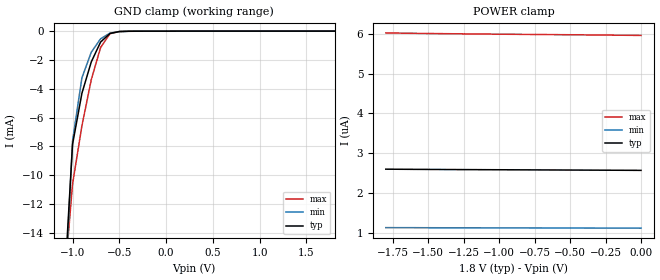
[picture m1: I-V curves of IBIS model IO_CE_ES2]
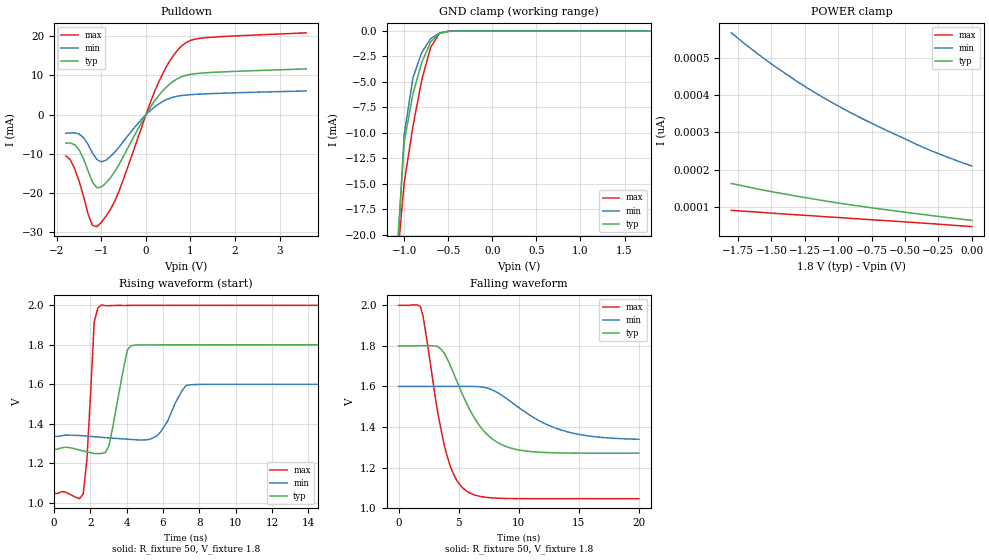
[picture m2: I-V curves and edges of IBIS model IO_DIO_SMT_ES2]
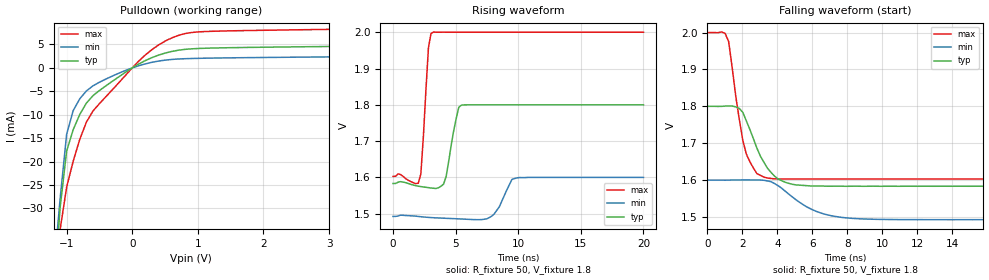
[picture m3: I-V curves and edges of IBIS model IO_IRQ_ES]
[IBIS Ver]   3.2
[Comment Char]   |_char
[File name]   r8900sa_18.ibs
[File Rev]   1.0
[Date]   2016/03/15
[Source]   This file orginated at SEIKO EPSON Corp.
[Notes]
[Disclaimer]
This information is for modeling purposes only, and is not guaranteed.
Property of SEIKO EPSON Corp.,
unauthorized reproduction and/or distribution is strictly prohibited.
[Copyright]
Copyright 2016, SEIKO EPSON Corp.
[Component]   r8900sa_18
Si_location Pin
Timing_location Pin
[Manufacturer]   SEIKO EPSON Corp.
[Package]
R_pkg   3.00m   NA   NA
L_pkg   3.70nH   NA   NA
C_pkg   0.70pF   NA   NA
[Pin] signal_name   model_name
1   CE   IO_CE_ES2
2   SCL   IO_INSPD2_ES2
3   FOUT   IO_OUT_ES
|4   N.C.
|5   VBAT   POWER2
6   VDD   POWER
7   FOE   IO_INSPD3_ES2
|8   N.C.
|9   N.C.
10   _INT   IO_IRQ_ES
11   VSS   POWER
|12   T2   TEST2
13   SDA   IO_DIO_SMT_ES2
| Models and submodels in the file (6): IO_CE_ES2 (Input), IO_DIO_SMT_ES2 (I/O_open_drain), IO_IRQ_ES (Open_drain), IO_INSPD3_ES2 (Input), IO_OUT_ES (3-state), IO_INSPD2_ES2 (Input)
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|14   N.C.
[Model]   IO_CE_ES2
Model_type Input
Enable Active-Low
Polarity Non-Inverting
Vinh=1.44
Vinl=0.36
C_comp   2.5p   2p   3p
[Temperature Range] 25   85   -40
[Voltage Range]   1.8   1.6   2.0
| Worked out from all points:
|   GND clamp passes 1 mA (typ) near -0.72 V on its own axis
[GND Clamp]
-1.8V     -154.7mA   -131.5mA   -191.9mA
-1.1V     -19.19mA   -20.8mA    -18.41mA
-1V       -7.861mA   -7.618mA   -10.62mA
-900mV    -4.316mA   -3.243mA   -6.579mA
-800mV    -2.138mA   -1.464mA   -3.37mA
-700mV    -753.3uA   -526.6uA   -1.13mA
-600mV    -160uA     -133.2uA   -178.7uA
-500mV    -27.2uA    -27.73uA   -23.08uA
-400mV    -6.23uA    -6.017uA   -7.112uA
1.8V      2.57uA     1.119uA    5.954uA
[POWER Clamp]
-1.8V     2.6uA      1.131uA    6.025uA
-1.7V     2.598uA    1.13uA     6.019uA
-1.6V     2.596uA    1.129uA    6.014uA
-1.5V     2.594uA    1.128uA    6.009uA
-1.3V     2.59uA     1.127uA    6.002uA
-1.1V     2.587uA    1.125uA    5.995uA
-400mV    2.577uA    1.121uA    5.975uA
-200mV    2.574uA    1.119uA    5.968uA
0V        2.57uA     1.118uA    5.961uA
[Model]   IO_DIO_SMT_ES2
Model_type I/O_open_drain
Enable Active-High
Polarity Non-Inverting
Vinh=1.44
Vinl=0.36
Vref=2.0
Vmeas=0.9
Rref=5000
C_comp   2.5p   2p   3p
[Temperature Range] 25   85   -40
[Voltage Range]   1.8   1.6   2.0
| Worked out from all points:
|   slope of the pulldown table from 0 to 0.27 V, typ, clamps not added: 58.7 ohm
|   GND clamp passes 1 mA (typ) near -0.69 V on its own axis
|   falling waveform, R_fixture 50, V_fixture 1.8: 20-80 % time 2.78ns typ, 4.41ns min, 1.74ns max; typ from 1.8 V to 1.27 V
|   rising waveform, R_fixture 50, V_fixture 1.8: 20-80 % time 637ps typ, 836ps min, 332ps max; typ from 1.27 V to 1.8 V
[Pulldown]
-1.8V     -7.266mA   -4.736mA   -10.53mA
-1.7V     -7.222mA   -4.672mA   -11.49mA
-1.5V     -9.036mA   -4.962mA   -17.01mA
-1.2V     -17.26mA   -9.79mA    -28.27mA
-1.1V     -18.67mA   -11.46mA   -28.53mA
-900mV    -17.42mA   -11.61mA   -25.92mA
-700mV    -14.52mA   -9.554mA   -22.05mA
-100mV    -2.011mA   -1.203mA   -3.294mA
300mV     5.046mA    2.816mA    8.649mA
800mV     9.634mA    4.854mA    17.49mA
1.3V      10.61mA    5.262mA    19.53mA
3.6V      11.64mA    6.027mA    20.83mA
[GND Clamp]
-1.8V     -198.9mA   -168.8mA   -245.1mA
-1.1V     -24.22mA   -25.62mA   -24.62mA
-1V       -10.89mA   -10.15mA   -14.91mA
-900mV    -6.13mA    -4.568mA   -9.309mA
-800mV    -3.058mA   -2.097mA   -4.786mA
-700mV    -1.078mA   -757.4uA   -1.604mA
-600mV    -224.6uA   -189.6uA   -244.1uA
-500mV    -33.81uA   -37.1uA    -22.82uA
-400mV    -4.624uA   -6.222uA   -2.07uA
1.8V      65pA       236.5pA    43.66pA
[POWER Clamp]
-1.8V     163.7pA    566.2pA    91.8pA
-1.6V     148.6pA    509.3pA    87.08pA
-1.4V     135.6pA    458.4pA    82.08pA
-1.2V     123.2pA    411.9pA    77.59pA
-1V       111.5pA    370.8pA    72.76pA
-800mV    101.2pA    333.3pA    67.98pA
-400mV    82.48pA    266pA      58.55pA
-200mV    73.47pA    236.5pA    53.66pA
0V        65.03pA    210.4pA    48.49pA
[Falling Waveform]
R_fixture=50
V_fixture=1.8
V_fixture_min=1.6
V_fixture_max=2.0
0s        1.8V       1.6V       2V
1.818ns   1.801V     1.6V       1.993V
3.232ns   1.797V     1.6V       1.48V
3.838ns   1.76V      1.6V       1.3V
4.646ns   1.655V     1.6V       1.159V
5.455ns   1.543V     1.6V       1.094V
7.273ns   1.368V     1.593V     1.053V
9.293ns   1.297V     1.527V     1.047V
13.74ns   1.272V     1.381V     1.047V
20ns      1.271V     1.34V      1.047V
[Rising Waveform]
R_fixture=50
V_fixture=1.8
V_fixture_min=1.6
V_fixture_max=2.0
0s        1.271V     1.336V     1.047V
1.616ns   1.262V     1.339V     1.045V
1.818ns   1.257V     1.338V     1.215V
2.222ns   1.249V     1.334V     1.915V
2.626ns   1.25V      1.331V     2.002V
3.03ns    1.287V     1.328V     1.998V
4.242ns   1.796V     1.32V      2V
5.657ns   1.8V       1.337V     2V
7.273ns   1.8V       1.594V     2V
20ns      1.8V       1.6V       2V
[Ramp]
R_load=50
dV/dt_r   3.176E-1/6.348E-10   1.584E-1/8.306E-10   5.721E-1/3.231E-10
dV/dt_f   3.175E-1/2.775E-9   1.563E-1/4.407E-9   5.720E-1/1.736E-9
|[End   IO_DIO_SMT_ES2
[Model]   IO_IRQ_ES
Model_type Open_drain
Enable Active-Low
Polarity Non-Inverting
Vref=2.0
Vmeas=0.9
Rref=5000
C_comp   2.5p   2p   3p
[Temperature Range] 25   85   -40
[Voltage Range]   1.8   1.6   2.0
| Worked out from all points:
|   slope of the pulldown table from 0 to 0.27 V, typ, clamps not added: 135 ohm
|   falling waveform, R_fixture 50, V_fixture 1.8: 20-80 % time 1.27ns typ, 2.06ns min, 790ps max; typ from 1.8 V to 1.58 V
|   rising waveform, R_fixture 50, V_fixture 1.8: 20-80 % time 653ps typ, 888ps min, 401ps max; typ from 1.58 V to 1.8 V
[Pulldown]
-1.8V     -181.8mA   -153.7mA   -225.3mA
-1.2V     -49.39mA   -44.1mA    -58.79mA
-1.1V     -29.93mA   -28mA      -34.58mA
-1V       -17.75mA   -14.17mA   -25.46mA
-900mV    -13.18mA   -9.113mA   -19.93mA
-800mV    -9.946mA   -6.599mA   -15.27mA
-700mV    -7.543mA   -4.939mA   -11.61mA
-600mV    -5.952mA   -3.846mA   -9.235mA
-400mV    -3.815mA   -2.373mA   -6.132mA
300mV     2.195mA    1.19mA     3.899mA
800mV     3.951mA    1.961mA    7.318mA
3.6V      4.668mA    2.416mA    8.354mA
[Falling Waveform]
R_fixture=50
V_fixture=1.8
V_fixture_min=1.6
V_fixture_max=2.0
0s        1.8V       1.6V       2V
1.01ns    1.801V     1.6V       1.998V
1.212ns   1.801V     1.6V       1.976V
1.818ns   1.794V     1.6V       1.765V
2.222ns   1.761V     1.6V       1.671V
3.232ns   1.648V     1.599V     1.608V
4.444ns   1.594V     1.57V      1.603V
6.061ns   1.584V     1.518V     1.603V
7.677ns   1.583V     1.499V     1.603V
20ns      1.583V     1.493V     1.603V
[Rising Waveform]
R_fixture=50
V_fixture=1.8
V_fixture_min=1.6
V_fixture_max=2.0
0s        1.583V     1.493V     1.603V
2.02ns    1.576V     1.492V     1.584V
2.222ns   1.575V     1.492V     1.61V
2.828ns   1.572V     1.49V      1.957V
3.232ns   1.57V      1.489V     2.001V
4.04ns    1.582V     1.488V     2V
5.455ns   1.799V     1.485V     2V
7.879ns   1.8V       1.493V     2V
9.899ns   1.8V       1.599V     2V
20ns      1.8V       1.6V       2V
[Ramp]
R_load=50
dV/dt_r   1.300E-1/6.461E-10   6.446E-2/8.883E-10   2.383E-1/3.825E-10
dV/dt_f   1.301E-1/1.262E-9   6.446E-2/2.055E-9   2.382E-1/7.718E-10
|[End   IO_IRQ_ES
